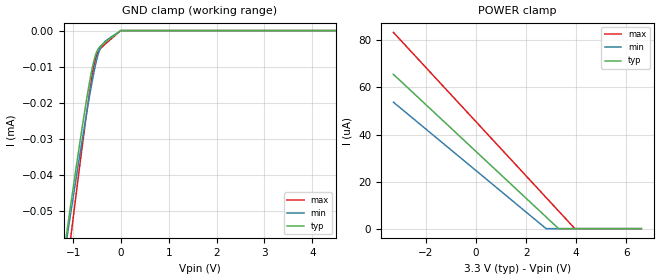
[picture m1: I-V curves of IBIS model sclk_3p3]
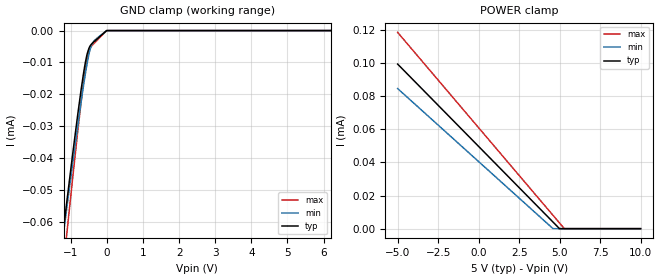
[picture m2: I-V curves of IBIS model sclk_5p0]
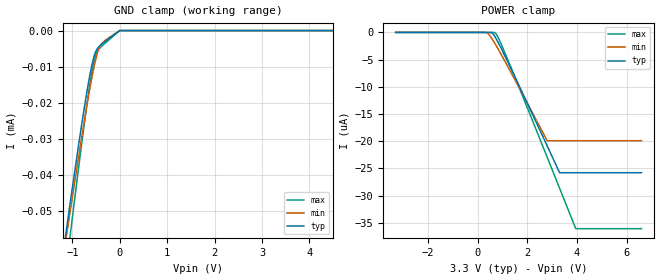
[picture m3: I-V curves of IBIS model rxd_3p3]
|Texas Instruments Incorporated
| PGA460-Q1 Ultrasonic Sensor Signal Conditioner
|Marketing part#   Digital Voltage Range   Package-type   #pins
| PGA460-Q1   2.8V-30V   TSSOP   16
[IBIS Ver]   4.1
[File name]   pga460-q1.ibs
[File Rev]   1.0
[Date]   02/14/2017
[Source]
| Texas Instruments Incorporated.
| Analog-eLab Design Center, HPA
| 12500 TI Blvd
| Dallas, TX -75243
[Notes]   Revision History:
| Rev 1.0: 02/14/2017
| - Initial version of the model
| - Model generated from simulations in SPECTRE
| - Model matched to SPICE simulation
| - C_comp although listed in numerical order of value are
|   obtained from varying PVT conditions. For PVT conditions for
|   each specific value refer the buffer description under
|   respective [Model]. IBIS model user is responsible for using
|   appropriate C_comp to simulate for Signal Integrity.
|* EXCEPTION:   *
|* - For sclk_* model,there is a leakage in Power clamp IV   *
|*   tables due to pullup resistor(RH1) connected to pad.   *
|* - For decpl model  Pullup and pulldown data donot cross zero   *
|*   due to Driver transistors(MN0 & MP0) connected to pad   *
|* - For decpl model Pullup and pulldown data donot cross zero   *
|*   due to Driver transistors(MN0 & MP0) connected to pad   *
|* - For io model there is a leakage in power clamp and ground clamp   *
|*   tables due to Resistor bank and driver transistor (MN_DIODE)   *
|*   connected to PAD   *
[Disclaimer]
| This model is designed as an aid for customers of Texas Instruments.
| TI and its licensors and suppliers make no warranties, either expressed
| or implied, with respect to this  model, including the warranties of
| merchantability or fitness for a particular purpose. The model is
| provided solely on an "as is" basis. The entire risk as to its quality
| and performance is with the customer.
[Copyright]
(C) Copyright 2017 Texas Instruments Incorporated.All rights reserved.
|   PGA460-Q1PW
[Component]   PGA460-Q1PW
[Manufacturer]   TI
[Package]   |16 TSSOP -PW package
|   typ   min   max
R_pkg   0.01   0.008   0.012
L_pkg   0.1nH   0.08nH   0.12nH
C_pkg   0.1pF   0.08pF   0.12pF
[Pin]  signal_name   model_name   R_pin   L_pin   C_pin
1   LIM   nc   NA   NA   NA
2   INP   nc   NA   NA   NA
3   INN   nc   NA   NA   NA
4   GND   power   NA   NA   NA
5   OUTA   nc   NA   NA   NA
6   GNDP   power   NA   NA   NA
7   OUTB   gnd   NA   NA   NA
8   IO   io   NA   NA   NA
9   TEST   nc   NA   NA   NA
10   TXD   txd   NA   NA   NA
11   RXD   rxd   NA   NA   NA
12   SCLK   sclk   NA   NA   NA
13   DECPL   decpl   NA   NA   NA
14   IOREG   power   NA   NA   NA
15   VPWR   power   NA   NA   NA
16   AVDD   power   NA   NA   NA
|   Model Selectors
[Model Selector] sclk
sclk_3p3   3.3V   digital Input
sclk_5p0   5.0V   digital Input
[Model Selector] rxd
rxd_3p3   3.3V   digital Input
rxd_5p0   5.0V   digital Input
[Model Selector] txd
txd_3p3   3.3V   digital Output
txd_5p0   5.0V   digital Output
[Model Selector] decpl
decpl_3p3   3.3V   digital Output
decpl_5p0   5.0V   digital Output
| Models and submodels in the file (9): sclk_3p3 (Input), sclk_5p0 (Input), rxd_3p3 (Input), rxd_5p0 (Input), txd_3p3 (Output), txd_5p0 (Output), decpl_3p3 (Output), decpl_5p0 (Output), io (I/O_open_drain)
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|   sclk_3p3 Model
[Model]   sclk_3p3
Model_type   Input
Vinl = 0.99
Vinh = 2.31
|   typ   min   max
|   (nom PVT)   (fast PVT)   (slow PVT)
C_comp   1.838e-13   1.828e-13   1.861e-13
| Where nom  PVT is Nominal Process, 3.3V, 27C
|   Fast PVT is Strong Process,  3.95V, -40C
|   Slow PVT is Weak Process,   2.8V, 125C
[Voltage Range]   3.3   2.8   3.95
|Junction Temperature
[Temperature Range]   27   125   -40
[Power Clamp Reference]   3.3   2.8   3.95
[GND Clamp Reference]   0   0   0
[GND Clamp]
|   Voltage   I(typ)   I(min)   I(max)
-3.3V     -269.7uA   -252.9uA   -308uA
-1.231V   -65.33uA   -66.49uA   -77.24uA
-1.06V    -49.38uA   -51.63uA   -58.66uA
-910.8mV  -35.73uA   -38.82uA   -42.68uA
-706.2mV  -18.17uA   -22.02uA   -21.88uA
-598.2mV  -10.32uA   -13.91uA   -12.35uA
-533.6mV  -6.898uA   -9.655uA   -8.076uA
-471.8mV  -5.023uA   -6.383uA   -5.776uA
-390.8mV  -3.877uA   -3.86uA    -4.469uA
-301.2mV  -2.962uA   -2.672uA   -3.422uA
-3.3mV    0A         0A         0A
6.6V      0A         0A         0A
[POWER Clamp]
|   Voltage   I(typ)   I(min)   I(max)
-3.3V     65.58uA    53.75uA    83.41uA
2.796V    4.982uA    14.1nA     13.24uA
3.297V    0A         0A         7.475uA
3.944V    0A         0A         20.14nA
6.6V      0A         0A         0A
|   sclk_5p0 Model
[Model]   sclk_5p0
Model_type   Input
Vinl = 1.5
Vinh = 3.5
|   typ   min   max
|   (nom PVT)   (fast PVT)   (slow PVT)
 C_comp   1.769e-13   1.741e-13   1.918e-13
| Where nom  PVT is Nominal Process, 5V, 27C
|   Fast PVT is Strong Process,  5.3V, -40C
|   Slow PVT is Weak Process,   4.6V, 125C
[Voltage Range]   5   4.6   5.3
|Junction Temperature
[Temperature Range]   27   125   -40
[Power Clamp Reference]   5   4.6   5.3
[GND Clamp Reference]   0   0   0
[GND Clamp]
|   Voltage   I(typ)   I(min)   I(max)
-5V       -442.4uA   -408uA     -501.1uA
-1.245V   -66.51uA   -67.58uA   -78.65uA
-1.154V   -57.98uA   -59.65uA   -68.73uA
-1.09V    -51.97uA   -54.04uA   -61.73uA
-929mV    -37.21uA   -40.21uA   -44.46uA
-717.6mV  -18.95uA   -22.77uA   -22.85uA
-616.9mV  -11.42uA   -15.12uA   -13.73uA
-542.7mV  -7.217uA   -10.1uA    -8.494uA
-464.4mV  -4.847uA   -5.99uA    -5.578uA
-386.2mV  -3.809uA   -3.74uA    -4.397uA
-5mV      0A         0A         -13.23nA
10V       0A         0A         0A
[POWER Clamp]
|   Voltage   I(typ)   I(min)   I(max)
-5V       99.36uA    84.58uA    118.5uA
4.596V    3.971uA    0A         8.047uA
4.995V    0A         0A         3.45uA
5.293V    0A         0A         24.17nA
10V       0A         0A         0A
|   rxd_3p3 Model
[Model]   rxd_3p3
Model_type   Input
Vinl = 0.99
Vinh = 2.1
|   typ   min   max
|   (nom PVT)   (fast PVT)   (slow PVT)
C_comp   1.864e-13   1.861e-13   1.876e-13
| Where nom  PVT is Nominal Process, 3.3V, 27C
|   Fast PVT is Strong Process,  3.95V, -40C
|   Slow PVT is Weak Process,   2.8V, 125C
[Voltage Range]   3.3   2.8   3.95
|Junction Temperature
[Temperature Range]   27   125   -40
[Power Clamp Reference]   3.3   2.8   3.95
[GND Clamp Reference]   0   0   0
[GND Clamp]
|   Voltage   I(typ)   I(min)   I(max)
-3.3V     -269.5uA   -252.7uA   -307.9uA
-1.234V   -65.53uA   -66.62uA   -77.49uA
-1.06V    -49.32uA   -51.52uA   -58.62uA
-910.8mV  -35.68uA   -38.73uA   -42.64uA
-706.2mV  -18.14uA   -21.94uA   -21.86uA
-598.2mV  -10.3uA    -13.85uA   -12.33uA
-533.6mV  -6.882uA   -9.602uA   -8.065uA
-471.8mV  -5.012uA   -6.337uA   -5.769uA
-390.8mV  -3.873uA   -3.822uA   -4.467uA
-301.2mV  -2.967uA   -2.645uA   -3.426uA
-1.75mV   -17.22nA   -1.302nA   0A
6.6V      0A         0A         0A
[POWER Clamp]
|   Voltage   I(typ)   I(min)   I(max)
-3.3V     65.87pA    64.69pA    157.5pA
286.8mV   6.953pA    -11.01nA   11.28pA
418.4mV   -325.9pA   -239.8nA   10.05pA
569.6mV   -83.49nA   -1.109uA   -143.1pA
716.1mV   -922nA     -2.194uA   -127.9nA
858mV     -2.119uA   -3.32uA    -1.236uA
1.169V    -4.988uA   -5.886uA   -4.514uA
2.801V    -20.85uA   -19.91uA   -22.93uA
3.303V    -25.78uA   -19.91uA   -28.65uA
3.952V    -25.78uA   -19.91uA   -36.07uA
6.6V      -25.78uA   -19.91uA   -36.07uA
